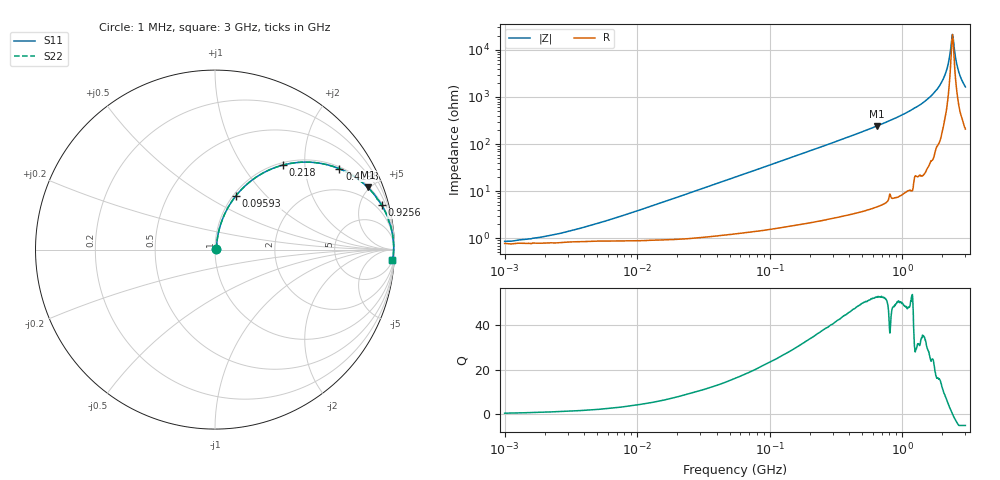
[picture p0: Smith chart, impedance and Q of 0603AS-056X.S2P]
!s-Parameter Generated by FASTRON Sdn. Bhd.
!FASTRON P/N : 0603AS-056X
!Keysight Technologies: E4991B_MY54100416_A.01.15
!Date created: Wed Oct 04 12:58:13 2023
!Version  : Rev01 Wed Oct 04 12:58:13 2023
!Data & Calibration Information:
!Freq	S11	S21	S12	S22
!PortZ  Port1:50+j0  Port2:50+j0
!When reading reference impedance value at option line is always used.
! Remarks : This data is being provided solely for informational purposes.
# Hz S dB R 50
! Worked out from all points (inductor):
!   1601 points, 1 MHz to 3 GHz, reference 50 ohm
!   read as one part in series: L = 59.1 nH near 7.075 MHz
!   highest Q = 52.4 at 648.8 MHz (marker M1), where L = 59.7 nH
!   self-resonance near 2.395 GHz
!   S11 on the Smith chart (normalised r, x): 1 MHz: 1.02, +0.01; 95.93 MHz: 1.03, +0.69; 218 MHz: 1.04, +1.55; 419.8 MHz: 1.07, +3.03; 925.6 MHz: 1.15, +7.49; 3 GHz: 5, -32
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1000000  -41.38 25.6  -0.07 -0.2  -0.07 -0.2  -41.38 25.6
1878552  -39.62 41.6  -0.07 -0.4  -0.07 -0.4  -39.62 41.6
3804036  -35.71 58.5  -0.07 -0.8  -0.07 -0.8  -35.71 58.5
1.447069e7  -25.42 77.3  -0.09 -3.0  -0.09 -3.0  -25.42 77.3
5.477226e7  -14.35 75.4  -0.27 -11.0  -0.27 -11.0  -14.35 75.4
9.593103e7  -9.89 68.8  -0.60 -18.7  -0.60 -18.7  -9.89 68.8
2.083556e8  -4.62 52.4  -2.02 -35.9  -2.02 -35.9  -4.62 52.4
2.179536e8  -4.37 51.2  -2.16 -37.2  -2.16 -37.2  -4.37 51.2
4.198105e8  -1.66 33.0  -5.26 -55.7  -5.26 -55.7  -1.66 33.0
6.488164e8  -0.73 22.2  -8.46 -66.7  -8.46 -66.7  -0.73 22.2
7.925923e8  -0.49 17.8  -10.30 -70.9  -10.30 -70.9  -0.49 17.8
9.255909e8  -0.34 14.9  -11.82 -74.0  -11.82 -74.0  -0.34 14.9
1.409185e9  -0.12 7.8  -17.34 -80.5  -17.34 -80.5  -0.12 7.8
1.855641e9  -0.05 3.7  -23.70 -82.8  -23.70 -82.8  -0.05 3.7
2.134733e9  -0.04 1.7  -30.40 -80.7  -30.40 -80.7  -0.04 1.7
2.221924e9  -0.04 1.1  -33.94 -77.2  -33.94 -77.2  -0.04 1.1
2.335937e9  -0.04 0.4  -41.70 -56.4  -41.70 -56.4  -0.04 0.4
2.39512e9  -0.04 0.0  -46.60 -5.6  -46.60 -5.6  -0.04 0.0
2.455801e9  -0.04 -0.3  -42.26 50.1  -42.26 50.1  -0.04 -0.3
2.581816e9  -0.05 -1.1  -34.04 73.1  -34.04 73.1  -0.05 -1.1
2.687267e9  -0.05 -1.7  -30.33 77.5  -30.33 77.5  -0.05 -1.7
3e9  -0.08 -3.4  -24.36 79.3  -24.36 79.3  -0.08 -3.4
